FUNCTION_BLOCK CheckXbotPos	//Rising edge triggered wrapper of the ReadXbotPox command
VAR_INPUT
	Execute : BOOL;	// Execution of the function block begins on a rising edge of this input.
	XbotID : USINT;	// xbot ID# (1-78)
END_VAR
VAR_OUTPUT
	Done : BOOL; // Execution successful. Function block is finished
	Valid : BOOL;	// xbot position is up-to-date, if false the output position is the last known position 
	PosX : REAL;	// xbot X position in meters
	PosY : REAL;	// xbot Y position in meters
	PosZ : REAL;	// xbot Z position in meters
	PosRx : REAL;	// xbot rotation about X axis in radians 
	PosRy : REAL;	// xbot rotation about Y axis in radians
	PosRz : Real;	// xbot rotation about Z axis in radians
END_VAR
VAR_IN_OUT
	PM_Controller : PMControllerType;	// the planar motor controller to use
END_VAR
VAR
	ReadXbotPos : PMC_ReadXbotPos;
END_VAR

IF(Execute = FALSE)THEN
	Done := FALSE;
	ReadXbotPos(Enable := FALSE,PM_Controller := PM_Controller);
END_IF;

IF(Execute = TRUE AND Done = FALSE)THEN
	Done := TRUE;
	ReadXbotPos(Enable := TRUE,XbotID := XbotID,Valid => Valid,PosX => PosX,PosY => PosY,PosZ => PosZ,PosRx => PosRx,PosRy => PosRy,PosRz => PosRz,PM_Controller := PM_Controller);
END_IF;

END_FUNCTION_BLOCK
